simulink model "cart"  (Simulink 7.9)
settings: Solver=ode23  StartTime=0.0  StopTime=3  RelTol=1e-6
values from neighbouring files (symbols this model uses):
  a_max = p0 = -    [assignment1.m]    (also in assignment3.m; assignment4.m)
  g = 9.81    [MPCsimulink.m]    (also in assignment4.m; pend_init.m; setupOptimization.m)
  g1 = c2d(tf([1 0],[tcAngleVel 1]),h,'tustin')    [assignment4.m]    (also in assignment5.m; pend_init.m)
  g2 = c2d(tf(1,[tcAngle 1]),h,'tustin')    [assignment4.m]    (also in assignment5.m; pend_init.m)
  g3 = c2d(tf(1),h)    [assignment1.m]    (also in assignment3.m = c2d(tf(1,[tcAcc 1]),h,'tustin'); assignment4.m = c2d(tf(1,[tcAcc 1]),h,'tustin'); assignment5.m = c2d(tf(1,[tcAcc 1]),h,'tustin'); pend_init.m = c2d(tf(1,[tcAcc 1]),h,'tustin'))
  h = uIn(5*N+10)    [MPCsimulink.m]    (also in pend_init.m = 0.01)
  initPendValue = [0;0]    [assignment3.m]    (also in assignment4.m; pend_init.m)
  initPosError = 0    [assignment1.m]    (also in assignment3.m; assignment4.m; assignment5.m; pend_init.m)
  l = 0.345    [MPCsimulink.m]    (also in assignment4.m; loaddym.m = fgetl(fid); pend_init.m)
  p0 = -0.8    [assignment5.m]
libraries: simulink x1

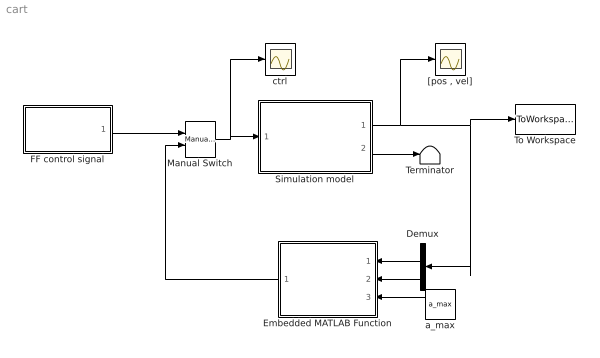
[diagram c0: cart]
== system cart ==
  Demux : Demux  Outputs=2
  Embedded MATLAB Function : MATLAB Function  TreatAsAtomicUnit=on
  FF control signal : Subsystem
  Manual Switch : simulink/Signal Routing/Manual Switch  sw=1  action=0  varsize=off
  Simulation model : Subsystem
  Terminator : Terminator
  To Workspace : ToWorkspace  VariableName=simout  SampleTime=-1  SaveFormat=Structure With Time
  "[pos , vel]" : Scope
  a_max : Constant  Value=a_max
  ctrl : Scope
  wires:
  Simulation model/1("[ pos [m] , vel [m/s] ]") -> "[pos , vel]"/1, To Workspace/1, Demux/1
  FF control signal/1(Out1) -> Manual Switch/1
  Manual Switch/1 -> ctrl/1, Simulation model/1(a_ref [m/s^2])
  Simulation model/2("[ ang [rad] , angVel [rad/s] ]") -> Terminator/1
  Embedded MATLAB Function/1(u) -> Manual Switch/2
  a_max/1 -> Embedded MATLAB Function/3(a_max)
  Demux/1 -> Embedded MATLAB Function/1(pos)
  Demux/2 -> Embedded MATLAB Function/2(vel)

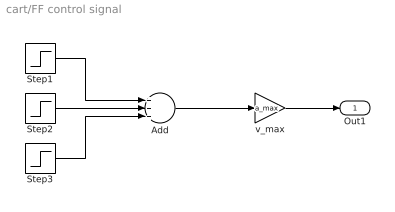
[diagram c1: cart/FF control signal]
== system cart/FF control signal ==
  Add : Sum  Inputs=+++
  Step1 : Step  Time=0  SampleTime=0
  Step2 : Step  Time=t(1)  After=-2  SampleTime=0
  Step3 : Step  Time=t(2)  SampleTime=0
  v_max : Gain  Gain=a_max  Multiplication=Matrix(K*u) (u vector)
  Out1 : Outport
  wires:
  Add/1 -> v_max/1
  v_max/1 -> Out1/1
  Step1/1 -> Add/1
  Step2/1 -> Add/2
  Step3/1 -> Add/3

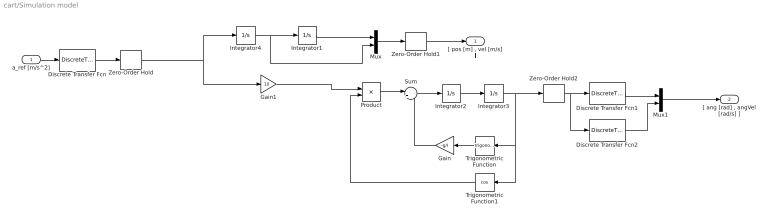
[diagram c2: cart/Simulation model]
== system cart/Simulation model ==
  a_ref [m/s^2] : Inport
  Discrete Transfer Fcn : DiscreteTransferFcn  Numerator=g3.num{1}  Denominator=g3.den{1}  SampleTime=h
  Discrete Transfer Fcn1 : DiscreteTransferFcn  Numerator=g2.num{1}  Denominator=g2.den{1}  SampleTime=h
  Discrete Transfer Fcn2 : DiscreteTransferFcn  Numerator=g1.num{1}  Denominator=g1.den{1}  SampleTime=h
  Gain : Gain  Gain=-g/l
  Gain1 : Gain  Gain=1/l
  Integrator1 : Integrator  InitialCondition=p0+initPosError
  Integrator2 : Integrator  InitialCondition=initPendValue(2)
  Integrator3 : Integrator  InitialCondition=initPendValue(1)
  Integrator4 : Integrator
  Mux : Mux  Inputs=2
  Mux1 : Mux  Inputs=2
  Product : Product
  Sum : Sum  Inputs=|++
  Trigonometric Function : Trigonometry
  Trigonometric Function1 : Trigonometry  Operator=cos
  Zero-Order Hold : ZeroOrderHold  SampleTime=h
  Zero-Order Hold1 : ZeroOrderHold  SampleTime=h
  Zero-Order Hold2 : ZeroOrderHold  SampleTime=h
  "[ pos [m] , vel [m/s] ]" : Outport
  "[ ang [rad] , angVel [rad/s] ]" : Outport  Port=2
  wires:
  Discrete Transfer Fcn/1 -> Zero-Order Hold/1
  Zero-Order Hold2/1 -> Discrete Transfer Fcn2/1, Discrete Transfer Fcn1/1
  Discrete Transfer Fcn2/1 -> Mux1/2
  Discrete Transfer Fcn1/1 -> Mux1/1
  Gain/1 -> Sum/2
  Trigonometric Function/1 -> Gain/1
  Trigonometric Function1/1 -> Product/2
  Product/1 -> Sum/1
  Gain1/1 -> Product/1
  a_ref [m/s^2]/1 -> Discrete Transfer Fcn/1
  Mux1/1 -> "[ ang [rad] , angVel [rad/s] ]"/1
  Mux/1 -> Zero-Order Hold1/1
  Sum/1 -> Integrator2/1
  Integrator3/1 -> Zero-Order Hold2/1, Trigonometric Function1/1, Trigonometric Function/1
  Integrator2/1 -> Integrator3/1
  Integrator1/1 -> Mux/1
  Integrator4/1 -> Mux/2, Integrator1/1
  Zero-Order Hold/1 -> Integrator4/1, Gain1/1
  Zero-Order Hold1/1 -> "[ pos [m] , vel [m/s] ]"/1

== matlab function Embedded
MATLAB Function ==
function u = fcn(pos,vel,a_max)
% pos is the position, vel is the velocity and a_max is a_max

% The if-clause is here to avoid chattering when close to the origin.
if ((pos/0.02)^2+(vel/0.1)^2>=0.3)
    u = 0;     % your controller goes here
else
    u = -3.12*pos-2.69*vel;  % to keep the cart at the origin, when close
end
